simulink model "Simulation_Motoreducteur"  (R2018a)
settings: Solver=VariableStepAuto  StartTime=0.0  StopTime=10.0  RelTol=1e-3
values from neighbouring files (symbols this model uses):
  r = 1/48    (= 0.0208333333333)    [Constantes.m]
libraries: fl_lib x7, nesl_utility x3, elec_lib x1, simulink x1

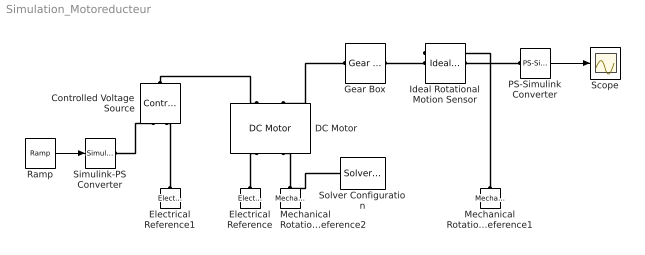
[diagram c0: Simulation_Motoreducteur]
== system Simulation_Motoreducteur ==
  Controlled Voltage Source : fl_lib/Electrical/Electrical Sources/Controlled Voltage Source
  DC Motor : elec_lib/Actuators & Drivers/Rotational Actuators/DC Motor  parameterization=1  Ra=r_induit Ohm  La=1.2e-5 H  emf_or_torque=1  Kv=k V/(rad/s)  Ki=6.876e-4 N*m/A  T_stall=2.4e-4 N*m  w_max=1.91e+4 rpm  w_rated=1.5e+4 rpm  P_rated=0.08 W  V_rated=1.5 V  J=1e-6 kg*m^2  lam_param=1  lam=1e-6 N*m/(rad/s)  i_noload=0 A  V_i_noload=1.5 V  speed0=0 rpm  alpha=0.00393 1/K  Tmeas=25 degC  thermal_mass=100 J/K  initial_temperature=25 degC
  Electrical Reference : fl_lib/Electrical/Electrical Elements/Electrical Reference
  Electrical Reference1 : fl_lib/Electrical/Electrical Elements/Electrical Reference
  Gear Box : fl_lib/Mechanical/Mechanisms/Gear Box  ratio=1/r  t_in_specify=off  t_in_priority=None  t_in=0 N*m  t_in_nominal_specify=off  t_in_nominal_unit=N*m  t_in_nominal_value=1  t_out_specify=off  t_out_priority=None  t_out=0 N*m  t_out_nominal_specify=off  t_out_nominal_unit=N*m  t_out_nominal_value=1
  Ideal Rotational Motion Sensor : fl_lib/Mechanical/Mechanical Sensors/Ideal Rotational Motion Sensor  offset=0 rad
  Mechanical Rotational Reference1 : fl_lib/Mechanical/Rotational Elements/Mechanical Rotational Reference
  Mechanical Rotational Reference2 : fl_lib/Mechanical/Rotational Elements/Mechanical Rotational Reference
  PS-Simulink Converter : nesl_utility/PS-Simulink Converter  PhysicalDomain=network_engine_domain  SubClassName=ps_output  LeftPortType=input  RightPortType=output  PseudoPeriodic=off  Frequencies=[]  Unit=1  AffineConversion=off
  Ramp : simulink/Sources/Ramp  slope=1  start=0  InitialOutput=0
  Scope : Scope
  Simulink-PS Converter : nesl_utility/Simulink-PS Converter  PhysicalDomain=network_engine_domain  SubClassName=ps_input  LeftPortType=input  RightPortType=output  PseudoPeriodic=off  Frequencies=[]  NoiseDistribution=none  NoiseParameters=[]  Unit=1  AffineConversion=off  FilteringAndDerivatives=provide  SimscapeFilterOrder=1  InputFilterTimeConstant=0.001  UdotUserProvided=0
  Solver Configuration : nesl_utility/Solver Configuration  PhysicalDomain=network_engine_domain  SubClassName=solver  LeftPortType=input  RightPortType=generic  Tones=[]  Harmonics=[]  SimulateNoise=off  Profile=off  UseLocalSampling=off  EnableSwitchedLinearOptims=on  FrequencyDomain=off  UseCCode=off  RelTol=0.001  AbsTol=1e-06  MinStep=1e-09  ToWorkspace=off  RevertToSquareIcSolve=off  NumHomotopyIterations=100  PhasorMode=off  PhasorModeNumHarmonics=1  DoDC=off  ResidualTolerance=1e-09  UseLocalSolver=off  LocalSolverChoice=NE_BACKWARD_EULER_ADVANCER  LocalSolverSampleTime=0.001  DoFixedCost=off  MaxNonlinIter=3  MaxModeIter=2  LinearAlgebra=Sparse  EquationFormulation=NE_TIME_EF  DelaysMemoryBudget=1024  AutomaticFiltering=on  FilteringTimeConstant=0.001
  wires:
  PS-Simulink Converter/1 -> Scope/1
  Ramp/1 -> Simulink-PS Converter/1
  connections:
  Electrical Reference/LConn1 -- DC Motor/RConn1
  Mechanical Rotational Reference2/LConn1 -- Solver Configuration/RConn1 -- DC Motor/RConn2
  Controlled Voltage Source/LConn1 -- DC Motor/LConn1
  Electrical Reference1/LConn1 -- Controlled Voltage Source/RConn2
  Gear Box/LConn1 -- DC Motor/LConn2
  Ideal Rotational Motion Sensor/RConn2 -- PS-Simulink Converter/LConn1
  Mechanical Rotational Reference1/LConn1 -- Ideal Rotational Motion Sensor/RConn1
  Ideal Rotational Motion Sensor/LConn1 -- Gear Box/RConn1
  Simulink-PS Converter/RConn1 -- Controlled Voltage Source/RConn1
